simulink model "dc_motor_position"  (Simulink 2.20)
settings: Solver=FixedStepDiscrete  StartTime=0.0  StopTime=.25  FixedStep=0.001  RelTol=1e-3  AbsTol=1e-6

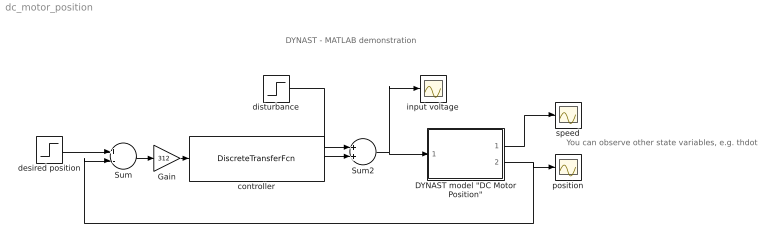
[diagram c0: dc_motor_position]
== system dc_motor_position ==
  note: DYNAST - MATLAB demonstration
  note: You can observe other state variables, e.g. thdot
  "DYNAST model \"DC Motor Position\"" : Subsystem
  Gain : Gain  Gain=312
  Sum : Sum  Inputs=+-
  Sum2 : Sum  Inputs=++
  controller : DiscreteTransferFcn  Numerator="[1.0000   -2.6500    2.3375   -0.6864]"  Denominator="[1.0000   -0.7200   -0.9660    0.6860]"  SampleTime=0.001
  desired position : Step  Time=0  Before=0  After=1
  disturbance : Step  Time=0  Before=0  After=0
  input voltage : Scope
  position : Scope
  speed : Scope
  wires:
  Sum/1 -> Gain/1
  Gain/1 -> controller/1
  "DYNAST model \"DC Motor Position\""/1(thetadot) -> speed/1
  controller/1 -> Sum2/2
  Sum2/1 -> "DYNAST model \"DC Motor Position\""/1(V), input voltage/1
  disturbance/1 -> Sum2/1
  desired position/1 -> Sum/1
  "DYNAST model \"DC Motor Position\""/2(theta) -> position/1, Sum/2

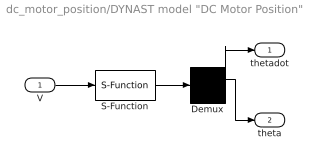
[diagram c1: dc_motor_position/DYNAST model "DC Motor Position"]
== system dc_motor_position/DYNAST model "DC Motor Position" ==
  V : Inport  Port=1  PortWidth=-1  SampleTime=-1
  Demux : Demux  Outputs=2
  S-Function : S-Function  FunctionName=dynPlantL  Parameters='%DYNAST%\examples\control\DCMotorPosition.prb',0.001  PortCounts=[]  SFunctionModules=''
  thetadot : Outport  Port=1
  theta : Outport  Port=2
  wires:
  V/1 -> S-Function/1
  S-Function/1 -> Demux/1
  Demux/2 -> thetadot/1
  Demux/1 -> theta/1
